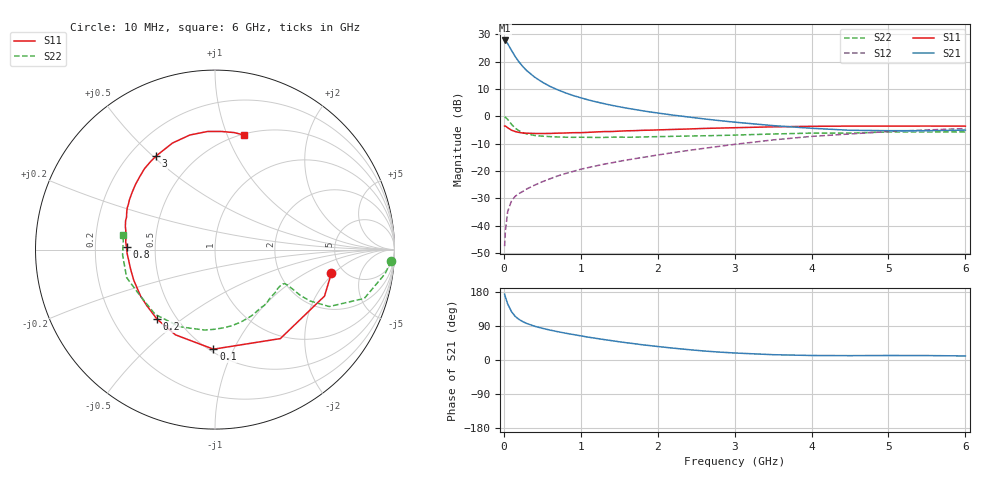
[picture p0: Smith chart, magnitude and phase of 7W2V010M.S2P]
! Infineon Technologies  Discrete & RF Semiconductors
! BFS17W
! Si NPN RF Bipolar Junction Transistor in SOT323
! VCE = 2 V  IC = 10 mA
! Common Emitter S-Parameters:  August  1999
# GHz  S  MA  R  50
!  f  S11  S21  S12  S22
! GHz  MAG  ANG  MAG  ANG  MAG  ANG  MAG  ANG
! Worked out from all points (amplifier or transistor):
!   36 points, 10 MHz to 6 GHz, reference 50 ohm
!   highest |S21| = 27.7 dB at 10 MHz (marker M1)
!   |S21| within 3 dB of that: start of sweep to 86.81 MHz
!   unconditionally stable (mu >= 1): 376.2 MHz to 2.943 GHz; 4.073 GHz to end of sweep
!   at 250 MHz: K = 0.82, MSG = 22.8 dB, |S12| = -27.5 dB
!   at 1.4 GHz: K = 1.25, MAG = 7.6 dB, |S12| = -17.1 dB
!   at 6 GHz: K = 1.09, MAG = -2.1 dB, |S12| = -4.5 dB
!   S11 on the Smith chart (normalised r, x): 10 MHz: 3.99, -1.87; 100 MHz: 0.52, -0.84; 200 MHz: 0.39, -0.41; 800 MHz: 0.34, +0.01; 3 GHz: 0.30, +0.51; 6 GHz: 0.51, +1.15
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0.01  0.6616 -11.5  24.3 173.5  0.0042 82.3  0.9835 -3.7
0.02  0.6629 -23.0  23.97 166.2  0.0078 83.3  0.9569 -8.1
0.05  0.6152 -53.7  21.2 147.9  0.0181 68.7  0.8753 -18.1
0.1  0.5549 -90.9  15.96 127.4  0.0284 55.9  0.7111 -26.5
0.15  0.5235 -114.9  12.19 114.7  0.0346 51.0  0.6011 -28.4
0.2  0.5044 -129.9  9.716 106.7  0.0387 51.8  0.5388 -28.2
0.25  0.4917 -140.6  8.003 100.8  0.0424 51.6  0.4974 -27.3
0.3  0.4886 -148.2  6.784 96.3  0.0469 53.7  0.4746 -26.7
0.4  0.4837 -159.5  5.189 89.1  0.0549 56.1  0.4447 -26.0
0.5  0.4827 -167.1  4.198 83.7  0.0633 58.6  0.4321 -26.1
0.6  0.4844 -172.6  3.514 79.0  0.0717 60.5  0.4234 -26.9
0.7  0.49 -177.5  3.041 74.8  0.0809 61.8  0.4174 -28.4
0.8  0.4932 178.5  2.679 70.8  0.0893 62.5  0.4136 -30.3
1.1  0.5074 168.3  1.984 60.2  0.1152 64.0  0.4106 -37.1
1.3  0.5233 162.2  1.701 54.0  0.1326 64.5  0.4096 -42.7
1.6  0.5414 154.6  1.402 45.4  0.1581 64.7  0.4122 -51.4
2.2  0.5733 140.4  1.048 31.3  0.2155 64.7  0.4288 -70.7
3  0.6163 122.1  0.779 18.5  0.3058 60.8  0.4519 -97.3
3.5  0.6393 111.7  0.673 14.0  0.3686 56.3  0.473 -114.6
4.5  0.6595 93.6  0.553 11.5  0.4736 43.9  0.4904 -148.7
5.5  0.6608 80.6  0.543 11.7  0.5606 31.7  0.5157 -176.7
6  0.6583 75.8  0.557 10.7  0.5947 25.9  0.5162 171.0
